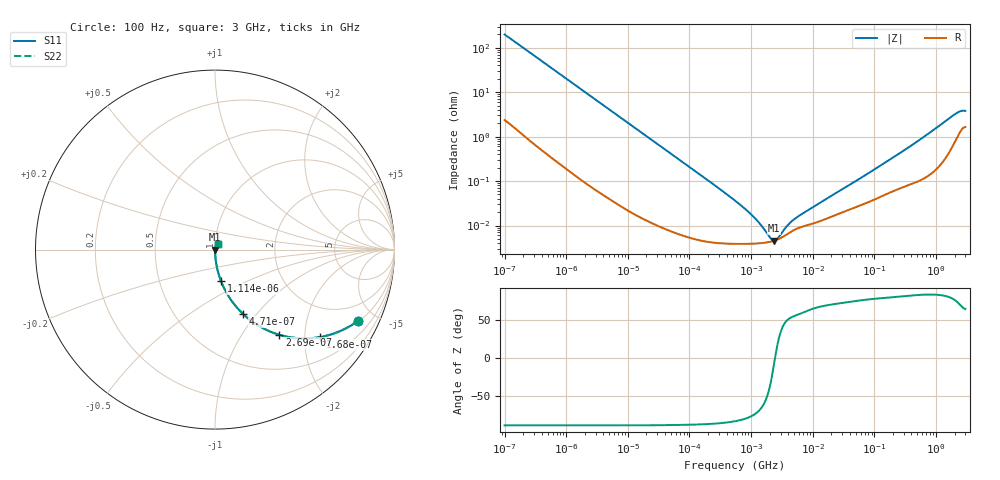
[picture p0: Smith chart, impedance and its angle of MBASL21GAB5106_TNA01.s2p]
! MBASL21GAB5106_TNA01  S-PARAMETER MODEL  ( Standard Model )
! Model Generated by TAIYO YUDEN Corporation (http://www.ty-top.com)
! Version 1.0
! TAIYO YUDEN Control No. 220601
! Copyright(c) 2012 TAIYO YUDEN CO.,LTD. All Rights Reserved.
! Product Description (link to TY-COMPAS)
! https://ds.yuden.co.jp/TYCOMPAS/or/detail?pn=MBASL21GAB5106KTNA01&u=M
! Products Name : Multilayer Ceramic Capacitors
! Characteristics :
!  Capacitance : 10 [uF] , Rated Voltage : 10 [V] , TCC : X5R
!  Case Size : 2.0 x 1.25 / 0.079 x 0.049 [mm/inch] , Thickness : 1.25 / 0.049 [mm/inch]
!  (Conditions: Temperature = 25 [degC] , DC Bias Voltage = 0 [V])
! External Node Assignments :
!  1  o---| |---o  2
! GND o---------o GND
! Frequency Range : 100Hz  -  3GHz  [ 401 STEP ]
# MHZ S RI R 50
! Freq[MHz].  S11 Real  S11 Imag  S21 Real  S21 Imag  S12 Real  S12 Imag  S22 Real  S22 Imag
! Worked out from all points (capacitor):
!   401 points, 100 Hz to 3 GHz, reference 50 ohm
!   read as one part in series: C = 7.99 uF near 109 Hz
!   lowest |Z| = 4.58 mohm at 2.367 MHz (marker M1)
!   series resonance near 2.449 MHz, so ESL is about 530 pH
!   S11 on the Smith chart (normalised r, x): 100 Hz: 1.05, -3.98; 168 Hz: 1.03, -2.38; 269 Hz: 1.02, -1.49; 471 Hz: 1.01, -0.85; 1.114 kHz: 1.00, -0.36; 3 GHz: 1.03, +0.07
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0.0001  0.7952 -0.3977  0.2048 0.3977  0.2048 0.3977  0.7952 -0.3977
0.000119  0.7351 -0.4355  0.2649 0.4355  0.2649 0.4355  0.7351 -0.4355
0.000168  0.5857 -0.4871  0.4143 0.4871  0.4143 0.4871  0.5857 -0.4871
0.000269  0.358 -0.4743  0.642 0.4743  0.642 0.4743  0.358 -0.4743
0.000471  0.1565 -0.3585  0.8435 0.3585  0.8435 0.3585  0.1565 -0.3585
0.000694  0.0799 -0.2665  0.9201 0.2665  0.9201 0.2665  0.0799 -0.2665
0.001114  0.0334 -0.175  0.9666 0.175  0.9666 0.175  0.0334 -0.175
0.001788  0.0137 -0.1116  0.9863 0.1116  0.9863 0.1116  0.0137 -0.1116
0.005476  0.00174 -0.0371  0.9983 0.0371  0.9983 0.0371  0.00174 -0.0371
0.031977  0.000137 -0.00643  0.9999 0.00643  0.9999 0.00643  0.000137 -0.00643
0.547723  3.87e-05 -0.000361  1 0.000361  1 0.000361  3.87e-05 -0.000361
0.918067  3.87e-05 -0.000195  1 0.000195  1 0.000195  3.87e-05 -0.000195
1.473992  4.02e-05 -9.04e-05  1 9.04e-05  1 9.04e-05  4.02e-05 -9.04e-05
2.366551  4.55e-05 -5.77e-06  1 5.77e-06  1 5.77e-06  4.55e-05 -5.77e-06
3.79959  6.29e-05 7.29e-05  0.9999 -7.29e-05  0.9999 -7.29e-05  6.29e-05 7.29e-05
5.597215  8.55e-05 0.00013  0.9999 -0.00013  0.9999 -0.00013  8.55e-05 0.00013
9.794414  0.000109 0.000228  0.9999 -0.000228  0.9999 -0.000228  0.000109 0.000228
175.1444  0.000552 0.00294  0.9994 -0.00294  0.9994 -0.00294  0.000552 0.00294
536.3016  0.00108 0.00829  0.9989 -0.00829  0.9989 -0.00829  0.00108 0.00829
2036.508  0.0086 0.0306  0.9914 -0.0306  0.9914 -0.0306  0.0086 0.0306
2525.516  0.0145 0.0341  0.9855 -0.0341  0.9855 -0.0341  0.0145 0.0341
3000  0.0173 0.0331  0.9827 -0.0331  0.9827 -0.0331  0.0173 0.0331
